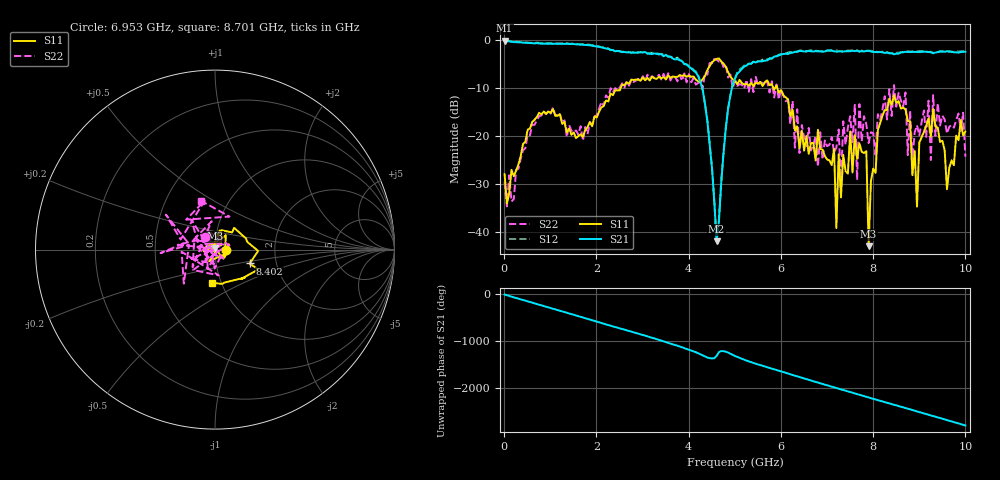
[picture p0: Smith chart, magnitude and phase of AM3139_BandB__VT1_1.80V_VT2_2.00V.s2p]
! Date/Time: Tue, Nov 13, 2018 4:59 PM
! Network Analyzer: Agilent Technologies E8364B Rev: A.07.50.67
! Sweep from 0.010 to 10.000 GHz, 201 Points, Sweep Type: LIN
! Power Supply: 1.801 V, 0.000 A
# Hz S DB R 50
!freq MagS11 AngS11 MagS21 AngS21 MagS12 AngS12 MagS22 AngS22
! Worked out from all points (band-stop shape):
!   201 points, 10 MHz to 10 GHz, reference 50 ohm
!   highest |S21| = -0.23 dB at 10 MHz (marker M1); lowest = -42.0 dB at 4.605 GHz (marker M2)
!   |S21| within 3 dB of the highest: start of sweep to 3.43 GHz; 5.968 GHz to end of sweep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
!   lowest |S11| = -43.0 dB at 7.902 GHz (marker M3), VSWR 1.01, Z = 49.9 + j0.693 ohm
!   |S11| at or under -10 dB: start of sweep to 2.532 GHz; 5.834 GHz to 5.881 GHz (46.62 MHz wide, 0.796 % of centre); 5.919 GHz to end of sweep
!   |S22| runs from -34.8 to -4.1 dB; largest |S21 - S12| = 0.026
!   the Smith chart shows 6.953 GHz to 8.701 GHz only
!   S11 on the Smith chart (normalised r, x): 6.953 GHz: 1.13, -0.01; 8.402 GHz: 1.46, -0.24; 8.701 GHz: 0.90, -0.35
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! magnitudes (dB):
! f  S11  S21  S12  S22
! 10 MHz  -28.0  -0.2  -0.2  -29.6
! 1.708 GHz  -20.3  -1.1  -1.0  -21.1
! 3.357 GHz  -7.8  -3.1  -3.0  -7.3
! 4.256 GHz  -8.9  -8.9  -8.8  -8.9
! 4.605 GHz  -4.0  -42.0  -42.0  -4.2
! 5.005 GHz  -8.5  -8.1  -8.0  -8.7
! 6.703 GHz  -21.5  -2.5  -2.3  -22.0
! 6.953 GHz  -24.3  -2.5  -2.4  -21.0
! 7.153 GHz  -22.8  -2.4  -2.2  -23.6
! 7.203 GHz  -39.3  -2.5  -2.3  -22.5
! 7.253 GHz  -23.9  -2.5  -2.4  -18.7
! 7.852 GHz  -23.3  -2.4  -2.3  -17.6
! 7.902 GHz  -43.0  -2.3  -2.3  -21.6
! 8.352 GHz  -12.4  -2.9  -2.9  -10.3
! 8.402 GHz  -13.6  -2.8  -2.9  -15.9
! 8.701 GHz  -14.6  -2.6  -2.6  -11.0
! 8.751 GHz  -17.0  -2.6  -2.4  -24.1
! 8.951 GHz  -34.8  -2.6  -2.5  -17.8
! 9.251 GHz  -20.2  -2.6  -2.5  -25.1
! 9.301 GHz  -14.5  -2.9  -2.7  -11.6
! 9.6 GHz  -31.2  -2.5  -2.4  -19.6
! 10 GHz  -19.2  -2.5  -2.4  -24.4
